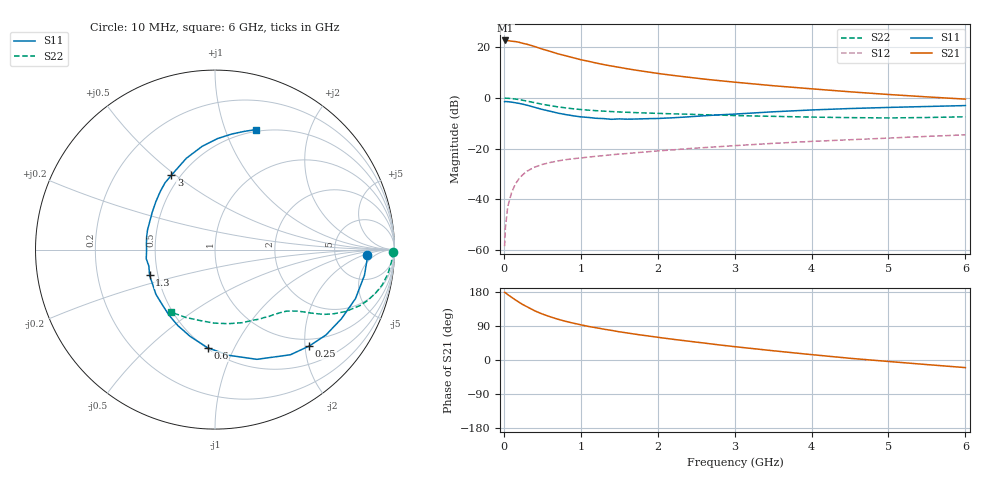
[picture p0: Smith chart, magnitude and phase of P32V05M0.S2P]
! SIEMENS Small Signal Semiconductors
! BFP181
! Si NPN RF Bipolar Junction Transistor in SOT143
! VCE = 2 V  IC = 5 mA
! Common Emitter S-Parameters:  March  1996
# GHz  S  MA  R  50
!  f  S11  S21  S12  S22
! GHz  MAG  ANG  MAG  ANG  MAG  ANG  MAG  ANG
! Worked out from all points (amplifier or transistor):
!   36 points, 10 MHz to 6 GHz, reference 50 ohm
!   highest |S21| = 22.7 dB at 20 MHz (marker M1)
!   |S21| within 3 dB of that: start of sweep to 459.9 MHz
!   unconditionally stable (mu >= 1): 1.592 GHz to end of sweep
!   at 250 MHz: K = 0.23, MSG = 25.8 dB, |S12| = -30.1 dB
!   at 1.4 GHz: K = 0.94, MSG = 17.5 dB, |S12| = -22.4 dB
!   at 6 GHz: K = 1.04, MAG = 5.8 dB, |S12| = -14.5 dB
!   lowest NFmin = 1.55 dB at 450 MHz
!   S11 on the Smith chart (normalised r, x): 10 MHz: 11, -2; 250 MHz: 0.85, -2.09; 600 MHz: 0.51, -0.79; 1.3 GHz: 0.45, -0.15; 3 GHz: 0.45, +0.48; 6 GHz: 0.48, +1.29
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0.01  0.8446 -2.0  13.48 178.6  0.0012 88.8  0.9897 -0.7
0.02  0.8487 -4.0  13.58 177.5  0.0027 88.3  0.9893 -1.7
0.05  0.845 -9.7  13.53 172.6  0.0071 85.5  0.9853 -4.1
0.15  0.8031 -28.6  12.91 158.6  0.0201 74.5  0.9527 -11.9
0.2  0.78 -37.6  12.48 152.1  0.0261 70.1  0.9264 -15.2
0.25  0.751 -45.7  11.89 145.9  0.0311 66.2  0.8978 -18.3
0.3  0.7208 -54.4  11.45 140.6  0.036 63.0  0.8674 -21.0
0.4  0.6543 -69.1  10.32 129.9  0.0433 56.7  0.8065 -25.3
0.5  0.5935 -82.7  9.172 121.4  0.0489 51.9  0.7517 -28.4
0.6  0.5483 -94.3  8.301 114.2  0.0534 48.7  0.7069 -30.7
0.7  0.5034 -105.9  7.433 107.8  0.0573 46.1  0.668 -32.3
0.8  0.4711 -116.1  6.806 102.2  0.0606 43.8  0.6378 -33.6
0.9  0.4457 -125.2  6.212 97.4  0.0634 42.4  0.6119 -34.7
1.1  0.4126 -143.0  5.276 88.6  0.0684 40.7  0.5749 -36.6
1.3  0.3917 -158.5  4.536 81.4  0.0732 39.3  0.5496 -38.5
1.7  0.3837 174.7  3.56 68.4  0.0829 38.3  0.5146 -42.4
2.2  0.4069 149.3  2.781 54.6  0.0949 37.0  0.486 -48.5
3  0.4808 120.3  2.048 35.2  0.1148 33.7  0.4497 -60.6
3.5  0.5334 107.4  1.742 24.4  0.1273 31.2  0.4342 -69.7
4.5  0.6187 88.7  1.322 4.5  0.1502 24.9  0.4094 -90.9
5.5  0.6785 76.1  1.049 -12.1  0.1748 19.3  0.4117 -113.4
6  0.7076 71.0  0.948 -20.1  0.1873 15.5  0.4253 -124.9
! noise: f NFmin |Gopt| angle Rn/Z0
0.45  1.55  0.48  17  0.36
0.9  1.65  0.4  35  0.34
1.8  2  0.18  88  0.34
